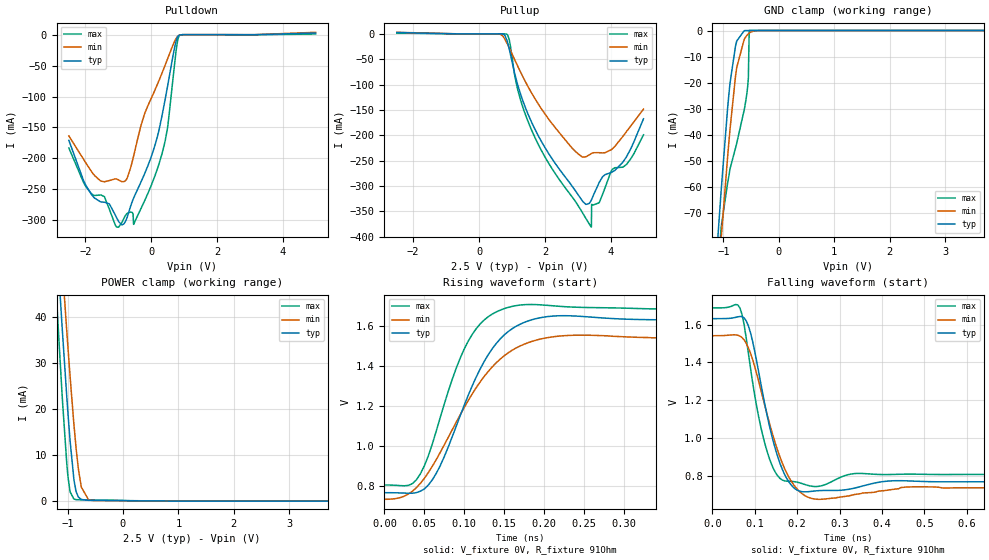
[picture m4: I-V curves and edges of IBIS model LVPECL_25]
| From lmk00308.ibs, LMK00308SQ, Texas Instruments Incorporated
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|   Model LVPECL_25
[Model]   LVPECL_25
Model_type   3-state
Polarity   Non-Inverting
Rref =   91.0000
Vmeas =   1.99
|   typ   min   max
|   Nom   Strong   Weak
C_comp   2.0749pF   1.9512pF   2.2734pF
|Output in low   Nom   Strong   Weak
|C_Comp   2.0749pF   1.9512pF   2.2734pF
|Output in High   Nom   Strong   Weak
|C_Comp   0.7651pF   0.6976pF   0.7651pF
[Voltage Range]   2.5   2.375   2.625
[Temperature Range]   45   125   -40
[Pullup Reference]   2.5   2.375   2.625
[Pulldown Reference]   -0   0   -0
[Power Clamp Reference]   2.5   2.375   2.625
[GND Clamp Reference]   0   -0   -0
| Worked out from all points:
|   slope of the pulldown table from 0 to 0.375 V, typ, clamps not added: 4.73 ohm
|   GND clamp passes 1 mA (typ) near -0.66 V on its own axis
|   POWER clamp passes 1 mA (typ) near -0.81 V on its own axis
|   falling waveform, V_fixture 0V, R_fixture 91Ohm: 20-80 % time 48.8ps typ, 60.3ps min, 41.4ps max; typ from 1.63 V to 0.768 V
|   rising waveform, V_fixture 0V, R_fixture 91Ohm: 20-80 % time 56ps typ, 71.7ps min, 45.7ps max; typ from 0.768 V to 1.63 V
[Pulldown]
|   Voltage   I(typ)   I(min)   I(max)
-2.5V     -170.9mA   -163.7mA   -183.2mA
-1.817V   -258mA     -220.8mA   -256.9mA
-1.42V    -270.8mA   -237.8mA   -261.8mA
-1.045V   -296.5mA   -233.4mA   -311.1mA
-880mV    -307.5mA   -237.7mA   -302.8mA
-625mV    -277.3mA   -215.2mA   -286.5mA
-535mV    -264.3mA   -196.5mA   -306.6mA
-205mV    -225.5mA   -128.7mA   -269.1mA
245mV     -152.3mA   -73.16mA   -207.5mA
492.5mV   -84.88mA   -39.88mA   -152mA
845mV     -1.078mA   -1.179mA   -2.211mA
4.992V    2.59mA     3.71mA     981.9uA
[GND Clamp]
|   Voltage   I(typ)   I(min)   I(max)
-2.5V     -680.7mA   -652.3mA   -694.7mA
-1.135V   -89.97mA   -107.4mA   -101.7mA
-1.045V   -62.74mA   -81.12mA   -76.76mA
-1.038V   -60.54mA   -78.99mA   -75.08mA
-925mV    -30mA      -48.72mA   -58.7mA
-880mV    -20.04mA   -37.72mA   -53.1mA
-760mV    -4.036mA   -14.22mA   -43.38mA
-625mV    -70.9uA    -3.386mA   -30.51mA
-572.5mV  -12.45uA   -1.77mA    -23.42mA
-550mV    -6.1uA     -1.283mA   -18.23mA
-535mV    -3.82uA    -1.017mA   0A
4.992V    0A         0A         0A
[Pullup]
|   Voltage   I(typ)   I(min)   I(max)
-2.5V     2.519mA    2.915mA    1.456mA
845mV     -12.71mA   -18.28mA   -985.4uA
1.167V    -99.82mA   -63.09mA   -109mA
1.58V     -172.3mA   -115.1mA   -187.8mA
2.84V     -301.8mA   -226.4mA   -322.9mA
3.245V    -336.5mA   -242.4mA   -364.4mA
3.41V     -327.6mA   -236.1mA   -381.3mA
3.417V    -326.6mA   -235.8mA   -336.4mA
3.65V     -292.8mA   -234.5mA   -332.6mA
4.032V    -272.8mA   -227.6mA   -268.4mA
4.475V    -242.6mA   -192.8mA   -257.7mA
4.992V    -167.7mA   -148.6mA   -199.2mA
[POWER Clamp]
|   Voltage   I(typ)   I(min)   I(max)
-2.5V     367mA      361.7mA    377.1mA
-1.21V    59.59mA    72.33mA    46.61mA
-1.143V   46.29mA    59.65mA    32.09mA
-1.105V   39.1mA     52.81mA    24.38mA
-1.09V    36.27mA    50.11mA    21.4mA
-1.015V   22.74mA    37.01mA    8.205mA
-955mV    13.09mA    27.12mA    2.027mA
-880mV    4.226mA    15.88mA    429.9uA
-805mV    886.5uA    6.959mA    296.1uA
-752.5mV  360.6uA    3.052mA    282.5uA
-595mV    172.5uA    235uA      254.5uA
4.992V    0A         0A         0A
[Ramp]
R_load = 91
|   typ   min   max
dV/dt_r   0.518031/5.60422e-11   0.48219/7.16356e-11   0.529005/4.56696e-11
dV/dt_f   0.518044/4.88422e-11   0.482317/6.01916e-11   0.528924/4.14467e-11
[Falling Waveform]
V_fixture = 0V
V_fixture_min = 0V
V_fixture_max = 0V
R_fixture = 91Ohm
C_fixture = 0F
|   Time   V(typ)   V(min)   V(max)
0s        1.631V     1.541V     1.688V
60ps      1.641V     1.543V     1.704V
80ps      1.619V     1.5V       1.526V
105ps     1.399V     1.335V     1.16V
125ps     1.163V     1.16V      960mV
170ps     808mV      839.7mV    772.7mV
200ps     723.2mV    729.1mV    765.5mV
250ps     720.4mV    674.6mV    743.2mV
340ps     736.6mV    701.6mV    811.6mV
1.39ns    767.8mV    735.5mV    806.5mV
[Rising Waveform]
V_fixture = 0V
V_fixture_min = 0V
V_fixture_max = 0V
R_fixture = 91Ohm
C_fixture = 0F
|   Time   V(typ)   V(min)   V(max)
0s        767.7mV    734.5mV    806.3mV
35ps      764.9mV    775mV      813mV
55ps      805.9mV    868.2mV    952.3mV
85ps      1.048V     1.083V     1.335V
105ps     1.255V     1.229V     1.526V
135ps     1.487V     1.396V     1.661V
165ps     1.6V       1.491V     1.703V
200ps     1.646V     1.54V      1.706V
245ps     1.649V     1.555V     1.694V
1.38ns    1.631V     1.539V     1.688V
